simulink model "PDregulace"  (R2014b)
settings: Solver=ode4  SolverMode=SingleTasking  StartTime=0.0  StopTime=30  FixedStep=0.001  RelTol=1e-3
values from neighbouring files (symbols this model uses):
  alfa = 0.2    [tlumeniPD.m]    (also in grafy.m = data(:,11); SITOrizeniPD.m; regulace1DoF.m = [4.65 9.06 15.39 13.86]; regulace2DoF.m = [4.65 9.06 15.39 13.86])
  dS = [parS(2)*parS(3)^2, (2*parS(4)*parS(2)*parS(3)+parS(3)^2), parS(2)+2*parS(4)*parS(3), 1]    [tlumeniPD.m]    (also in tlumeniP.m)
  Kp = -6    [tlumeniPD.m]    (also in SITOrizeniP.m = -4.5; SITOrizeniPD.m = -4; tlumeniP.m = -8)
  parS = [-0.0628 0.17 0.22 0.0318]    [tlumeniPD.m]    (also in tlumeniP.m)
  Td = 0.3    [tlumeniPD.m]    (also in SITOrizeniPD.m = 0.005)
libraries: simulink x2

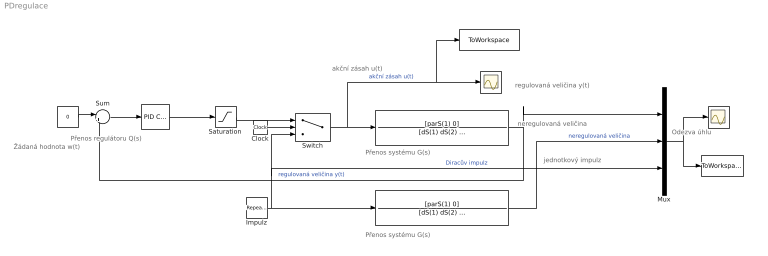
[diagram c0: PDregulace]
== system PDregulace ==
  note: Odezva úhlu
  note: neregulovaná veličina
  note: jednotkový impulz
  note: akční zásah u(t)
  note: Přenos systému G(s)
  note: Přenos systému G(s)
  note: Přenos regulátoru Q(s)
  note: Žádaná hodnota w(t)
  note: regulovaná veličina y(t)
  "  " : Constant  Value=0
  "    " : simulink/Continuous/PID Controller  Controller=PID  TimeDomain=Continuous-time  SampleTime=-1  IntegratorMethod=Forward Euler  FilterMethod=Forward Euler  Form=Parallel  P=Kp  I=0  D=Td*Kp  N=1/(alfa*Td)  InitialConditionSource=internal  InitialConditionForIntegrator=0  InitialConditionForFilter=0  ExternalReset=none  LimitOutput=off  UpperSaturationLimit=inf  LowerSaturationLimit=-inf  LinearizeAsGain=on  AntiWindupMode=none  Kb=1  TrackingMode=off  Kt=1  PParamMin=[]  PParamMax=[]  IParamMin=[]  IParamMax=[]  DParamMin=[]  DParamMax=[]  NParamMin=[]  NParamMax=[]  KbParamMin=[]  KbParamMax=[]  KtParamMin=[]  KtParamMax=[]  POutMin=[]  POutMax=[]  IOutMin=[]  IOutMax=[]  DOutMin=[]  DOutMax=[]  NOutMin=[]  NOutMax=[]  KbOutMin=[]  KbOutMax=[]  KtOutMin=[]  KtOutMax=[]  IntegratorOutMin=[]  IntegratorOutMax=[]  FilterOutMin=[]  FilterOutMax=[]  SumOutMin=[]  SumOutMax=[]  SumI1OutMin=[]  SumI1OutMax=[]  SumI2OutMin=[]  SumI2OutMax=[]  SumI3OutMin=[]  SumI3OutMax=[]  SumDOutMin=[]  SumDOutMax=[]  SaturationOutMin=[]  SaturationOutMax=[]  IntegratorContinuousStateAttributes=''  IntegratorStateMustResolveToSignalObject=off  IntegratorRTWStateStorageClass=Auto  FilterContinuousStateAttributes=''  FilterStateMustResolveToSignalObject=off  FilterRTWStateStorageClass=Auto  DifferentiatorICPrevScaledInput=0  DifferentiatorOutMin=[]  DifferentiatorOutMax=[]  UseFilter=on
  "     " : TransferFcn  Numerator=[parS(1) 0]  Denominator=[dS(1) dS(2) dS(3) dS(4)]
  "         " : Scope
  "                         " : TransferFcn  Numerator=[parS(1) 0]  Denominator=[dS(1) dS(2) dS(3) dS(4)]
  "                                 " : ToWorkspace  VariableName=dataPreg  SaveFormat=Timeseries  SampleTime=-1
  "                                           " : Scope
  "                                                                                  " : ToWorkspace  VariableName=akcniZasahPreg  SaveFormat=Timeseries  SampleTime=-1
  Clock : Clock
  Impulz : simulink/Sources/Repeating Sequence  rep_seq_t=[0 2.99 3 3.99 4 40]  rep_seq_y="[0  0     1   1    0      0]"
  Mux : Mux  Inputs=3
  Saturation : Saturate  UpperLimit=1  LowerLimit=-1
  Sum : Sum  Inputs=|+-
  Switch : Switch  Threshold=8
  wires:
  "  "/1 -> Sum/1
  "     "/1 -> Sum/2, Mux/1  "regulovaná veličina y(t)"
  "    "/1 -> Saturation/1
  Sum/1 -> "    "/1
  Impulz/1 -> "                         "/1, Mux/3, Switch/3  "Diracův impulz"
  Mux/1 -> "                                 "/1, "         "/1
  Switch/1 -> "                                           "/1, "                                                                                  "/1, "     "/1  "akční zásah u(t)"
  Saturation/1 -> Switch/1
  Clock/1 -> Switch/2
  "                         "/1 -> Mux/2  "neregulovaná veličina"
